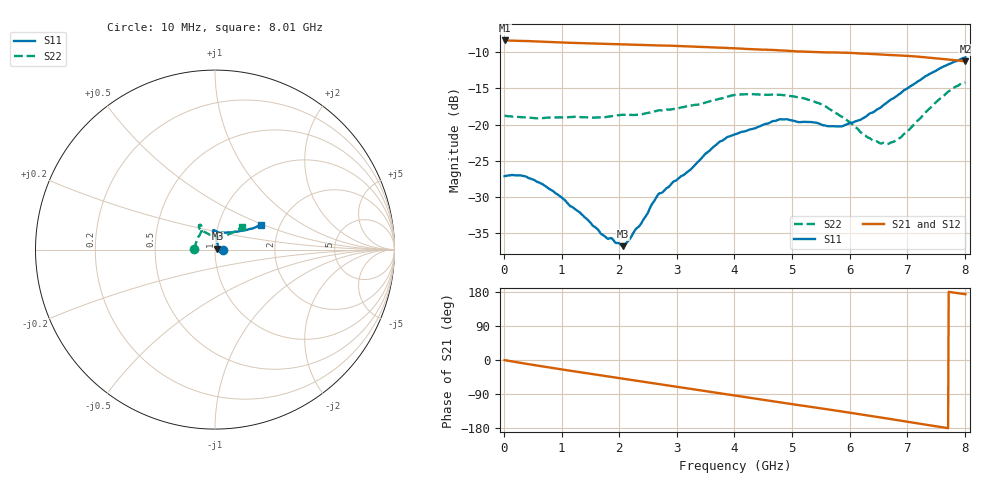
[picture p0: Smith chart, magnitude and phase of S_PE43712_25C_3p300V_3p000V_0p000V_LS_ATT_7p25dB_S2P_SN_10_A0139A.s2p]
! DEVICE ID: PE43712
! File Path: z:\PE43713\PE43713_CHAR_NOM_04292014\AMB\3p300\LS_ATT_7p25dB\PE43713_AMB_3p300V_3p000V_0p000V_LS_ATT_7p25dB_S2P_SN_10_A0139A.s2p
! Serial: 10
! Lot: A0139A
! Temp: 25C
! VDD: 3.300
! VSS: 0.000
! Control_Hi: 3.000
! Control_Lo: 0.000
! Attenuation Step: 7.25dB
! Port 1: RF1
! Port 2: RF2
! ThroughPath:1-2
! IDD: 0.0001475491
! ISS: -1.221e-007
#  Hz  S  RI  R  50
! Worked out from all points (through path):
!   801 points, 10 MHz to 8.01 GHz, reference 50 ohm
!   highest |S21| = -8.40 dB at 10 MHz (marker M1); lowest = -11.3 dB at 8.01 GHz (marker M2)
!   group delay of S21, straight-line fit = 64 ps
!   lowest |S11| = -36.8 dB at 2.07 GHz (marker M3), VSWR 1.03, Z = 51.4 + j0.576 ohm
!   |S11| at or under -10 dB: start of sweep to end of sweep
!   |S22| runs from -22.7 to -14.2 dB; largest |S21 - S12| = 0.0013
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1e7  0.0442 -5.85e-05  0.3803 -0.00217  0.3803 -0.00204  -0.1155 0.000701
3.3e8  0.0437 -0.00774  0.3728 -0.0564  0.3725 -0.056  -0.1119 0.0109
6.3e8  0.0377 -0.0116  0.359 -0.1028  0.3591 -0.1029  -0.1089 0.02
9.6e8  0.03 -0.0122  0.3374 -0.1495  0.3376 -0.1495  -0.1079 0.0302
1.35e9  0.0222 -0.00934  0.3061 -0.1978  0.3061 -0.1979  -0.1044 0.042
1.71e9  0.0172 -0.00283  0.2718 -0.2375  0.2719 -0.2375  -0.098 0.055
2.07e9  0.0134 0.00561  0.2328 -0.2719  0.2328 -0.2718  -0.0944 0.0689
2.38e9  0.0138 0.0156  0.1952 -0.2965  0.1952 -0.2964  -0.0851 0.0813
2.68e9  0.0156 0.0293  0.1571 -0.3142  0.1571 -0.3143  -0.0769 0.0991
3.23e9  0.00822 0.048  0.082 -0.3359  0.0821 -0.336  -0.0732 0.1134
3.72e9  0.00355 0.0748  0.015 -0.3391  0.0148 -0.339  -0.0749 0.1298
4.01e9  -0.00165 0.0858  -0.0245 -0.3348  -0.0245 -0.3348  -0.0823 0.1374
4.79e9  -0.00888 0.1086  -0.1207 -0.3016  -0.1207 -0.3019  -0.09 0.133
5.35e9  0.00262 0.1038  -0.1783 -0.2621  -0.1782 -0.2619  -0.0867 0.1179
5.63e9  0.0146 0.0964  -0.2034 -0.2399  -0.2034 -0.24  -0.0728 0.1069
5.88e9  0.0282 0.0936  -0.2264 -0.2168  -0.2258 -0.2168  -0.0562 0.0978
6.18e9  0.0525 0.094  -0.2479 -0.1849  -0.2474 -0.185  -0.0314 0.0838
6.4e9  0.0745 0.0957  -0.2609 -0.1606  -0.2604 -0.1605  -0.0122 0.0768
6.68e9  0.1071 0.0981  -0.274 -0.1272  -0.2737 -0.1272  0.0167 0.072
6.99e9  0.1426 0.1039  -0.2841 -0.0891  -0.2838 -0.0891  0.0463 0.0755
7.7e9  0.2267 0.125  -0.2814 -0.00194  -0.2811 -0.0022  0.1259 0.1103
8.01e9  0.2562 0.1378  -0.2714 0.0303  -0.2709 0.0298  0.1493 0.1262
